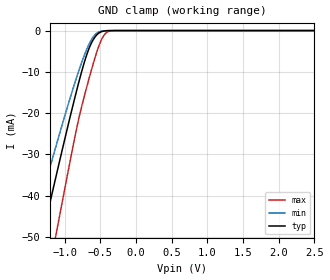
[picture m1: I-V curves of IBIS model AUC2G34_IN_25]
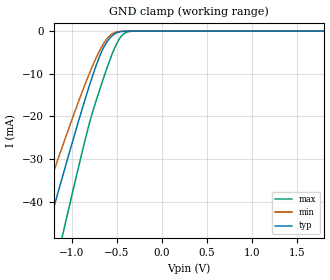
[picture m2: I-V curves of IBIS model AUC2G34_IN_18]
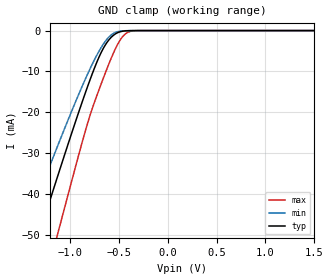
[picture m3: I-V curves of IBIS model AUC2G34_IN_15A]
| TEXAS INSTRUMENTS INCORPORATED
| Standard Linear and Logic Group
| IBIS Model of SN74AUC2G34
| Dual Buffer Gate
| This file contains package information for the following:
|  SOT 6-pin (DBV) package as [Component] AUC2G34_DBV
|  SOT 6-pin (DCK) package as [Component] AUC2G34_DCK
|  DSBGA 6-pin (YEP) package as [Component] AUC2G34_YEP
|  DSBGA 6-pin (YZP) package as [Component] AUC2G34_YZP
|  DSBGA 6-pin (YZT) package as [Component] AUC2G34_YZT
| This device can be powered at the following Vccs:
|  2.5 volt Vcc
|  1.8 volt Vcc
|  1.5 volt Vcc
|  1.2 volt Vcc
|  0.8 volt Vcc
| This file provides unique models under the [Model Selector] for each Vcc.
| For operation at a specific Vcc, select the appropriate model after each
| [Model Selector] keyword.
[IBIS Ver]   3.2
[Comment char]  |_char
[File Name]   sn74auc2g34.ibs
[File Rev]   1.3 | x_die
[Date]   November 21, 2003
[Source]   Data created from TI-SPICE simulations at TI-SLL.
[Notes]   The following is an IBIS list for the AUC2G34.
   Please contact sllibis@ti.com with questions and
   comments concerning SLL IBIS models.
   FILE REV HISTORY
   - 1.3 YZT package added to IBIS file on 12/19/07
   - Power-clamp data has been deleted since there is no
   power-clamp diode in the device.
   - Non-monotonic data in pullup and pulldown due to
   feedback circuit.
   - End point warning due to AC and DC mismatch.
[Disclaimer] Property of Texas Instruments Incorporated.  Unauthorized
   reproduction and/or distribution is strictly prohibited.
   This product is protected under copyright law.
   Created  2002, (C) Copyright  2002, Texas Instruments
   Incorporated, All Rights Reserved
   UNLESS THERE IS A SIGNED, WRITTEN AGREEMENT TO THE
   CONTRARY, TEXAS INSTRUMENTS (TI) IS PROVIDING THE IBIS
   MODELS  AND WITHOUT ANY WARRANTY, EXPRESSED OR
   IMPLIED.  TI assumes no liability for:
   1) the accuracy of the IBIS models provided to your
   company;
   2) the proper functioning of these IBIS Models in your
   design or for any resulting applications; or
   3) infringement of patents, copyrights or intellectual
   property rights resulting from your use of these IBIS
   models.
   TI provides IBIS Models as a service to our customers.
   You and your company shall not distribute, sell or give
   these models to anyone else without prior written
   permission from TI.
   TI reserves the right to make changes to our products or
   to discontinue any semiconductor product or service
   without notice, and advises our customers to obtain the
   latest version of relevant information to verify, before
   placing orders, that the information being relied on is
   current.
   Please be aware that your receipt and use of the IBIS
   information provided shall serve as acceptance of these
   terms and conditions.  If you do not accept these terms,
   you should return or destroy the IBIS models and any
   other accompanying information immediately.
| Component AUC2G34_DCK 6-pin SOT
[Component]   AUC2G34_DCK
[Manufacturer]   Texas Instruments, Inc.
[Package]
|   typ   min   max
R_pkg   1.400e-02   1.100e-02   2.100e-02
L_pkg   9.480e-10   7.840e-10   1.103e-09
C_pkg   1.910e-13   1.670e-13   2.050e-13
[Pin]   signal_name   model_name   R_pin   L_pin   C_pin
1   A1   AUC2G34_IN   1.300e-02   9.840e-10   1.960e-13
2   GND   GND   2.100e-02   1.103e-09   2.050e-13
3   A2   AUC2G34_IN   1.100e-02   9.980e-10   1.970e-13
4   Y2   AUC2G34_OUT   1.300e-02   9.040e-10   1.900e-13
5   VCC   POWER   1.500e-02   7.840e-10   1.670e-13
6   Y1   AUC2G34_OUT   1.200e-02   9.160e-10   1.950e-13
| Component AUC2G34_DBV 6-pin SOT
[Component]   AUC2G34_DBV
[Manufacturer]   Texas Instruments, Inc.
[Package]
|   typ   min   max
R_pkg   0.025   0.019   0.037
L_pkg   1.524nH   1.260nH   1.751nH
C_pkg   0.245pF   0.198pF   0.264pF
[Pin]   signal_name   model_name   R_pin   L_pin   C_pin
1   1A   AUC2G34_IN   0.021   1.405nH   0.246pF
2   GND   GND   0.037   1.751nH   0.263pF
3   2A   AUC2G34_IN   0.026   1.493nH   0.247pF
4   2Y   AUC2G34_OUT   0.019   1.620nH   0.264pF
5   VCC   POWER   0.024   1.260nH   0.198pF
6   1Y   AUC2G34_OUT   0.021   1.617nH   0.250pF
| Component AUC2G34_YEP 6-pin DSBGA
[Component]   AUC2G34_YEP
[Manufacturer]   Texas Instruments, Inc.
[Package]
|   typ   min   max
R_pkg   1.000e-03   1.000e-03   1.000e-03
L_pkg   2.460e-11   2.400e-11   2.500e-11
C_pkg   6.500e-14   6.400e-14   6.700e-14
[Pin]   signal_name   model_name   R_pin   L_pin   C_pin
1   1A   AUC2G34_IN   1.000e-03   2.500e-11   6.400e-14
2   GND   GND   1.000e-03   2.400e-11   6.700e-14
3   2A   AUC2G34_IN   1.000e-03   2.500e-11   6.400e-14
4   2Y   AUC2G34_OUT   1.000e-03   2.500e-11   6.400e-14
5   VCC   POWER   1.000e-03   2.400e-11   6.700e-14
6   1Y   AUC2G34_OUT   1.000e-03   2.500e-11   6.400e-14
| Component AUC2G34_YZP 6-pin DSBGA
[Component]   AUC2G34_YZP
[Manufacturer]   Texas Instruments, Inc.
[Package]
|   typ   min   max
R_pkg   1.000e-03   1.000e-03   1.000e-03
L_pkg   2.460e-11   2.400e-11   2.500e-11
C_pkg   6.500e-14   6.400e-14   6.700e-14
[Pin]   signal_name   model_name   R_pin   L_pin   C_pin
1   1A   AUC2G34_IN   1.000e-03   2.500e-11   6.400e-14
2   GND   GND   1.000e-03   2.400e-11   6.700e-14
3   2A   AUC2G34_IN   1.000e-03   2.500e-11   6.400e-14
4   2Y   AUC2G34_OUT   1.000e-03   2.500e-11   6.400e-14
5   VCC   POWER   1.000e-03   2.400e-11   6.700e-14
6   1Y   AUC2G34_OUT   1.000e-03   2.500e-11   6.400e-14
| Component AUC2G34_YZT 6-pin DSBGA
[Component]   AUC2G34_YZT
[Manufacturer]   Texas Instruments, Inc.
[Package]
|   typ   min   max
R_pkg   1.000e-03   1.000e-03   1.000e-03
L_pkg   2.460e-11   2.400e-11   2.500e-11
C_pkg   6.500e-14   6.400e-14   6.700e-14
[Pin]   signal_name   model_name   R_pin   L_pin   C_pin
1   1A   AUC2G34_IN   1.000e-03   2.500e-11   6.400e-14
2   GND   GND   1.000e-03   2.400e-11   6.700e-14
3   2A   AUC2G34_IN   1.000e-03   2.500e-11   6.400e-14
4   2Y   AUC2G34_OUT   1.000e-03   2.500e-11   6.400e-14
5   VCC   POWER   1.000e-03   2.400e-11   6.700e-14
6   1Y   AUC2G34_OUT   1.000e-03   2.500e-11   6.400e-14
| Model AUC2G34_IN
[Model Selector]   AUC2G34_IN
AUC2G34_IN_25   2.5 volt Vcc
AUC2G34_IN_18   1.8 volt Vcc
AUC2G34_IN_15A   1.5 volt Vcc
AUC2G34_IN_12   1.2 volt Vcc
AUC2G34_IN_08   0.8 volt Vcc
| Model AUC2G34_OUT
[Model Selector]   AUC2G34_OUT
AUC2G34_OUT_25   2.5 volt Vcc
AUC2G34_OUT_18   1.8 volt Vcc
AUC2G34_OUT_15A   1.5 volt Vcc
AUC2G34_OUT_12   1.2 volt Vcc
AUC2G34_OUT_08   0.8 volt Vcc
| Models and submodels in the file (10): AUC2G34_IN_25 (Input), AUC2G34_IN_18 (Input), AUC2G34_IN_15A (Input), AUC2G34_IN_12 (Input), AUC2G34_IN_08 (Input), AUC2G34_OUT_25 (Output), AUC2G34_OUT_18 (Output), AUC2G34_OUT_15A (Output), AUC2G34_OUT_12 (Output), AUC2G34_OUT_08 (Output)
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[Model]   AUC2G34_IN_25
Model_type  Input
Vinl=0.7
Vinh=1.7
| variable   typ   min   max
C_comp   2.34pF   1.88pF   2.74pF
[Temperature Range]   40   100   -40
| Ambient temperature   25   85   -40
[Voltage range]   2.5   2.3   2.7
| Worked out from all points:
|   GND clamp passes 1 mA (typ) near -0.55 V on its own axis
[GND Clamp]
| AUC2G34_IN_25
|   Voltage   I(typ)   I(min)   I(max)
-3.6V     -226.6mA   -190.3mA   -271.8mA
-1.455V   -60.71mA   -48.79mA   -79.87mA
-1.295V   -48.52mA   -38.74mA   -65.35mA
-1.105V   -34.25mA   -27.09mA   -48.1mA
-850mV    -15.85mA   -12.35mA   -25.34mA
-785mV    -11.51mA   -8.949mA   -20.15mA
-725mV    -7.81mA    -6.074mA   -16.01mA
-625mV    -3.071mA   -2.25mA    -9.633mA
-520mV    -618.6uA   -332uA     -3.783mA
-430mV    -73.2uA    -35.47uA   -776.9uA
-325mV    -3.339uA   -2.035uA   -30.74uA
2.5V      313.9pA    402pA      470.4pA
[Model]   AUC2G34_IN_18
Model_type  Input
Vinl=0.5775
Vinh=1.2675
| variable   typ   min   max
C_comp   2.41pF   1.97pF   2.74pF
[Temperature Range]   40   100   -40
| Ambient temperature   25   85   -40
[Voltage range]   1.8   1.65   1.95
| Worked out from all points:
|   GND clamp passes 1 mA (typ) near -0.55 V on its own axis
[GND Clamp]
| AUC2G34_IN_18
|   Voltage   I(typ)   I(min)   I(max)
-3.6V     -226.6mA   -190.3mA   -271.8mA
-1.435V   -59.19mA   -47.53mA   -78.05mA
-1.26V    -45.87mA   -36.57mA   -62.17mA
-1.105V   -34.25mA   -27.09mA   -48.1mA
-1.08V    -32.4mA    -25.59mA   -45.83mA
-810mV    -13.15mA   -10.23mA   -22.06mA
-685mV    -5.638mA   -4.364mA   -13.41mA
-565mV    -1.378mA   -858.8uA   -6.102mA
-490mV    -325.9uA   -162.9uA   -2.495mA
-425mV    -63.96uA   -31.11uA   -688.8uA
-300mV    -1.501uA   -1.001uA   -11.88uA
1.8V      203.2pA    298.4pA    235.5pA
[Model]   AUC2G34_IN_15A
Model_type  Input
Vinl=0.49
Vinh=1.04
| variable   typ   min   max
C_comp   2.45pF   2.01pF   2.75pF
[Temperature Range]   40   100   -40
| Ambient temperature   25   85   -40
[Voltage range]   1.5   1.4   1.6
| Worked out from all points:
|   GND clamp passes 1 mA (typ) near -0.55 V on its own axis
[GND Clamp]
| AUC2G34_IN_15A
|   Voltage   I(typ)   I(min)   I(max)
-3.6V     -226.6mA   -190.3mA   -271.8mA
-1.465V   -61.48mA   -49.43mA   -80.77mA
-1.29V    -48.15mA   -38.43mA   -64.9mA
-1.13V    -36.11mA   -28.6mA    -50.37mA
-1.08V    -32.4mA    -25.59mA   -45.83mA
-815mV    -13.48mA   -10.49mA   -22.45mA
-695mV    -6.152mA   -4.773mA   -14.06mA
-575mV    -1.605mA   -1.034mA   -6.664mA
-500mV    -407.2uA   -207.5uA   -2.896mA
-435mV    -83.64uA   -40.42uA   -873uA
-310mV    -2.072uA   -1.331uA   -17.49uA
1.5V      165.9pA    259.7pA    172.1pA
